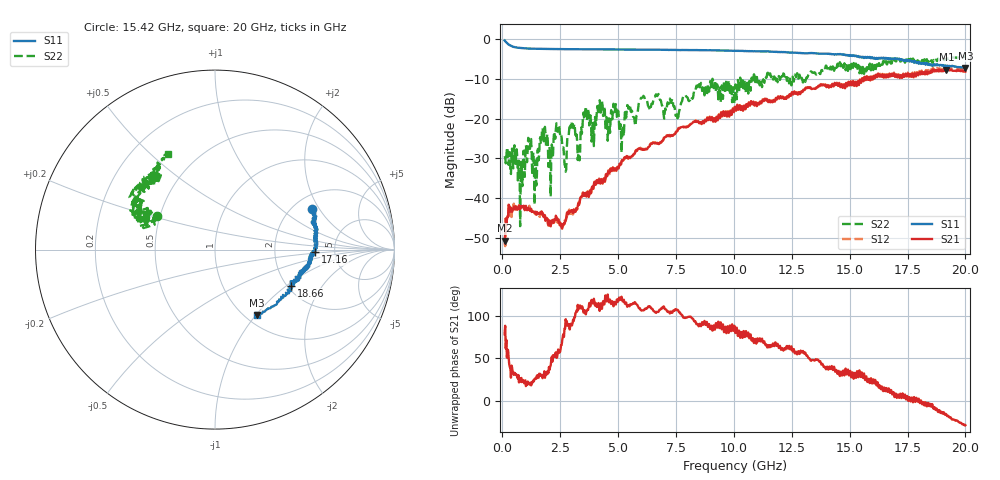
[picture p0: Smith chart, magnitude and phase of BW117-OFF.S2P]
!  2-Port S-parameters saved by WinCal
! VAR MeasName=S-Parameters (CALIBRATED_DATA) read from VNA (N5244A)
! VAR MeasDate=11/28/2011 3:35:24 PM
! VAR NAME=240-1 2
! VAR FILENAME=240-1 2.S2P
! VAR DATE=11/28/2011 3:35:24 PM
! VAR PHYS_PORTS=1,2
! VAR ObjTypeName=DATASET
! VAR IndexType=Frequency
# Hz S MA R 50
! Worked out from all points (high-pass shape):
!   801 points, 100 MHz to 20 GHz, reference 50 ohm
!   highest |S21| = -7.71 dB at 19.18 GHz (marker M1); lowest = -50.6 dB at 100 MHz (marker M2)
!   |S21| within 3 dB of the highest: 15.42185 GHz to 15.47161 GHz (49.76 MHz wide, 0.322 % of centre); 15.51 GHz to end of sweep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
!   lowest |S11| = -7.3 dB at 20 GHz (marker M3), VSWR 2.52, Z = 56.5 - j50.6 ohm
!   |S11| at or under -10 dB: nowhere
!   |S22| runs from -47.0 to -4.5 dB; largest |S21 - S12| = 0.027
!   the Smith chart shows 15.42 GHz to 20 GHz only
!   S11 on the Smith chart (normalised r, x): 15.42 GHz: 2.52, +1.73; 17.16 GHz: 3.51, -0.15; 18.66 GHz: 2.10, -1.09; 20 GHz: 1.13, -1.01
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1e8  0.9556 -42.6  0.002938 78.8  0.002805 73.1  0.03375 -9.2
3.985e8  0.8143 -115.5  0.006883 41.5  0.005804 33.0  0.03661 -10.6
7.71625e8  0.7682 -148.8  0.007289 22.5  0.007495 22.5  0.004454 -55.3
1.14475e9  0.7564 -164.7  0.007267 20.6  0.007414 21.0  0.05587 -58.1
1.468125e9  0.7514 -173.6  0.006191 25.9  0.00663 24.8  0.01444 -78.4
1.74175e9  0.7479 -179.5  0.00655 26.5  0.006715 30.0  0.07574 -64.3
2.09e9  0.7459 174.1  0.004432 41.6  0.005064 46.8  0.01045 -72.6
2.363625e9  0.7458 169.8  0.005355 50.9  0.005733 47.6  0.08064 -83.0
2.687e9  0.7433 165.0  0.004748 85.5  0.005454 80.9  0.02666 -104.0
2.9855e9  0.7419 161.0  0.007085 90.1  0.006827 91.3  0.08202 -72.7
3.43325e9  0.7406 155.4  0.01041 111.6  0.01062 111.4  0.0644 -62.9
4.22925e9  0.7397 145.7  0.01522 110.2  0.01526 109.6  0.1485 -110.6
5.149625e9  0.7354 135.6  0.02891 123.3  0.02853 123.3  0.03724 -123.6
6.741625e9  0.7314 118.6  0.04805 105.3  0.04834 105.2  0.2033 -137.1
1.005e10  0.7063 84.6  0.1405 84.0  0.1426 83.7  0.2136 -133.3
1.338325e10  0.6634 48.9  0.2357 48.3  0.2388 48.0  0.378 -179.2
1.5423e10  0.5873 22.6  0.2928 35.8  0.295 35.7  0.3705 150.1
1.669162e10  0.5599 6.7  0.3371 14.4  0.3438 14.4  0.4814 145.7
1.716425e10  0.5574 -1.5  0.3217 4.7  0.3306 4.6  0.5574 138.4
1.865675e10  0.4711 -25.4  0.391 -7.8  0.4085 -9.1  0.529 127.3
1.917912e10  0.4528 -35.5  0.4116 -16.7  0.4256 -17.9  0.5487 124.8
2e10  0.4325 -57.3  0.388 -29.4  0.4099 -31.3  0.5948 116.2
